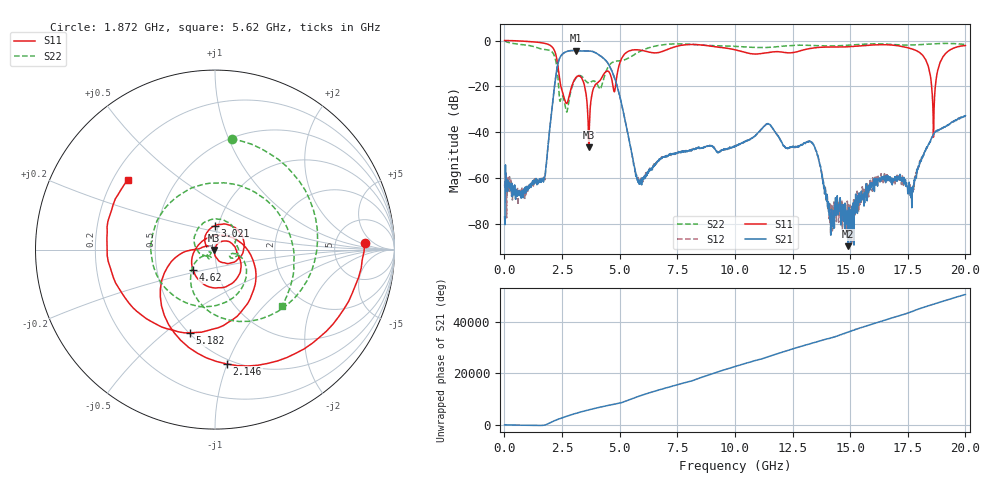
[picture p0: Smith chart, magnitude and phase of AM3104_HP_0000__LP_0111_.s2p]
!Created with skrf (http://scikit-rf.org).
# Hz S RI R 50.0
!freq ReS11 ImS11 ReS21 ImS21 ReS12 ImS12 ReS22 ImS22
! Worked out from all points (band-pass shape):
!   1601 points, 10 MHz to 20 GHz, reference 50 ohm
!   highest |S21| = -4.37 dB at 3.121 GHz (marker M1); lowest = -89.9 dB at 14.9 GHz (marker M2)
!   |S21| within 3 dB of the highest: 2.415 GHz to 4.252 GHz (1.837 GHz wide, 55.1 % of centre)
!   lowest |S11| = -46.7 dB at 3.658 GHz (marker M3), VSWR 1.01, Z = 49.6 - j0.256 ohm
!   |S11| at or under -10 dB: 2.307 GHz to 5.002 GHz (2.696 GHz wide, 73.8 % of centre); 18.34 GHz to 18.89 GHz (541 MHz wide, 2.91 % of centre)
!   |S22| runs from -31.3 to -0.2 dB; largest |S21 - S12| = 0.0045
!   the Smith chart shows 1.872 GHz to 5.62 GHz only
!   S11 on the Smith chart (normalised r, x): 1.872 GHz: 10, +3; 2.146 GHz: 0.46, -1.00; 3.021 GHz: 0.96, +0.26; 4.62 GHz: 0.76, -0.18; 5.182 GHz: 0.51, -0.61; 5.62 GHz: 0.26, +0.33
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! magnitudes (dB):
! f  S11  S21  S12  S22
! 10 MHz  0.0  -77.1  -63.7  -0.2
! 1.659 GHz  -1.1  -60.8  -61.0  -3.8
! 1.872 GHz  -1.6  -48.2  -48.0  -4.1
! 2.146 GHz  -3.9  -22.4  -22.4  -6.2
! 2.671 GHz  -27.3  -4.9  -4.9  -30.3
! 3.021 GHz  -17.5  -4.4  -4.4  -17.9
! 3.121 GHz  -16.0  -4.4  -4.3  -16.2
! 3.346 GHz  -16.2  -4.6  -4.6  -15.6
! 3.658 GHz  -46.7  -4.6  -4.6  -18.6
! 4.62 GHz  -15.5  -12.4  -12.3  -10.0
! 5.182 GHz  -6.3  -32.3  -32.3  -8.6
! 5.62 GHz  -4.1  -54.5  -53.7  -6.3
! 6.682 GHz  -5.3  -52.7  -52.4  -2.1
! 10.01 GHz  -4.0  -46.1  -45.9  -2.6
! 13.34 GHz  -3.3  -44.7  -44.7  -2.2
! 14.18 GHz  -2.9  -76.8  -71.4  -2.3
! 14.9 GHz  -2.8  -89.9  -75.6  -2.1
! 16.68 GHz  -1.9  -60.2  -61.1  -1.6
! 17.65 GHz  -3.6  -64.2  -65.9  -2.0
! 18.61 GHz  -42.2  -41.1  -41.1  -1.4
! 19.01 GHz  -7.3  -38.1  -38.3  -1.3
! 20 GHz  -2.2  -32.8  -33.0  -1.7
